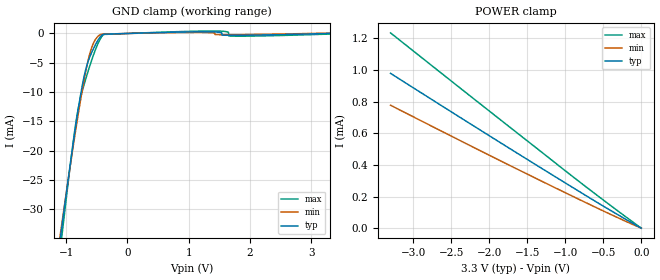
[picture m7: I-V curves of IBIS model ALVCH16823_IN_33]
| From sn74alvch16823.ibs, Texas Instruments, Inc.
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[Model]   ALVCH16823_IN_33
Model_type  Input
Vinl=0.8
Vinh=2.145
| variable   typ   min   max
C_comp   2.59pF   1.80pF   3.18pF
[Temperature Range]   40   100   -40
| Ambient temperature   25   85   -40
[Voltage range]   3.3   3   3.6
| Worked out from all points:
|   GND clamp passes 1 mA (typ) near -0.47 V on its own axis
[GND Clamp]
| ALVCH16823_IN_33
|   Voltage   I(typ)   I(min)   I(max)
-3.3V     -222.6mA   -207.9mA   -245.6mA
-1.125V   -37.48mA   -36.6mA    -39.69mA
-1.065V   -32.7mA    -32.19mA   -34.28mA
-880mV    -18.51mA   -19.03mA   -18.25mA
-795mV    -12.54mA   -13.36mA   -12.47mA
-700mV    -7.074mA   -7.617mA   -8.518mA
-605mV    -3.802mA   -3.189mA   -5.285mA
-440mV    -556.5uA   -200.5uA   -900.1uA
-375mV    -121.9uA   -99.83uA   -161.9uA
1.165V    276.8uA    180.6uA    398.2uA
1.715V    -314.2uA   -207.1uA   -457.4uA
3.3V      46.64pA    64.32uA    -103.1uA
[POWER Clamp]
| ALVCH16823_IN_33
|   Voltage   I(typ)   I(min)   I(max)
-3.3V     978.4uA    777uA      1.234mA
-1.29V    371.9uA    292.1uA    472.6uA
-645mV    181.5uA    142.1uA    231.1uA
-48.03fV  46.64pA    149pA      50.72pA
